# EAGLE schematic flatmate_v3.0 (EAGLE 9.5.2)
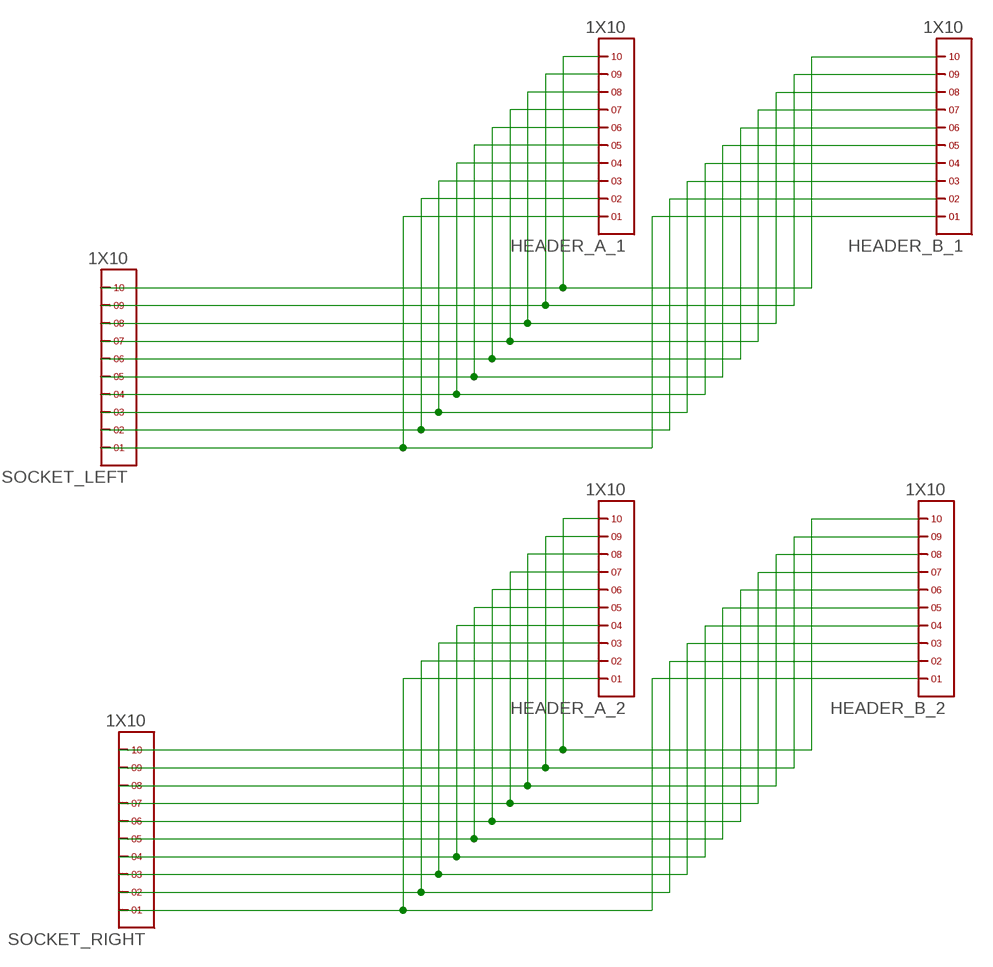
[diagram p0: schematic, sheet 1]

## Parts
HEADER_A_1  1X10  [1X10]
HEADER_A_2  1X10  [1X10]
HEADER_B_1  1X10  [1X10]
HEADER_B_2  1X10  [1X10]
SOCKET_LEFT  1X10  [1X10]
SOCKET_RIGHT  1X10  [1X10]

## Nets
N$1: HEADER_A_1.1 HEADER_B_1.1 SOCKET_LEFT.1
N$2: HEADER_A_1.2 HEADER_B_1.2 SOCKET_LEFT.2
N$3: HEADER_A_1.3 HEADER_B_1.3 SOCKET_LEFT.3
N$4: HEADER_A_1.5 HEADER_B_1.5 SOCKET_LEFT.5
N$5: HEADER_A_1.4 HEADER_B_1.4 SOCKET_LEFT.4
N$6: HEADER_A_2.1 HEADER_B_2.1 SOCKET_RIGHT.1
N$7: HEADER_A_1.6 HEADER_B_1.6 SOCKET_LEFT.6
N$8: HEADER_A_2.2 HEADER_B_2.2 SOCKET_RIGHT.2
N$9: HEADER_A_2.3 HEADER_B_2.3 SOCKET_RIGHT.3
N$10: HEADER_A_1.7 HEADER_B_1.7 SOCKET_LEFT.7
N$11: HEADER_A_2.4 HEADER_B_2.4 SOCKET_RIGHT.4
N$12: HEADER_A_2.5 HEADER_B_2.5 SOCKET_RIGHT.5
N$13: HEADER_A_1.8 HEADER_B_1.8 SOCKET_LEFT.8
N$14: HEADER_A_2.6 HEADER_B_2.6 SOCKET_RIGHT.6
N$15: HEADER_A_2.7 HEADER_B_2.7 SOCKET_RIGHT.7
N$16: HEADER_A_1.9 HEADER_B_1.9 SOCKET_LEFT.9
N$17: HEADER_A_2.8 HEADER_B_2.8 SOCKET_RIGHT.8
N$18: HEADER_A_2.9 HEADER_B_2.9 SOCKET_RIGHT.9
N$19: HEADER_A_1.10 HEADER_B_1.10 SOCKET_LEFT.10
N$20: HEADER_A_2.10 HEADER_B_2.10 SOCKET_RIGHT.10

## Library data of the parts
HEADER_A_1 HEADER_A_2 HEADER_B_1 HEADER_B_2 SOCKET_LEFT SOCKET_RIGHT = crazyflie:1X10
